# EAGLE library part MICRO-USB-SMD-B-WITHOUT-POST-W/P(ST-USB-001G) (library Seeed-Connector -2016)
320010000
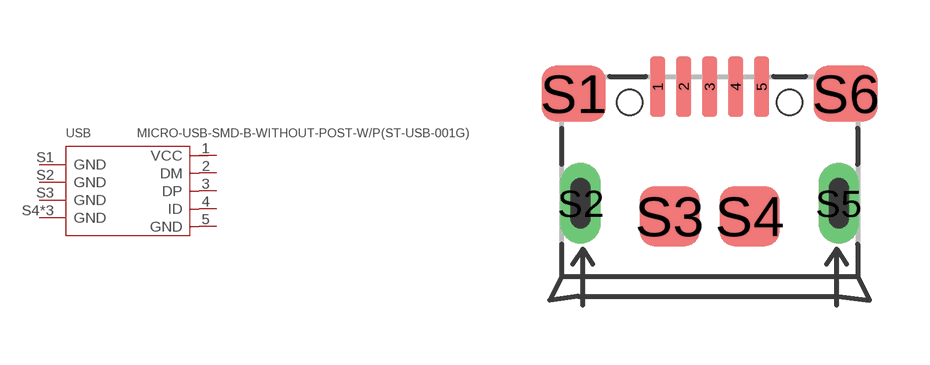
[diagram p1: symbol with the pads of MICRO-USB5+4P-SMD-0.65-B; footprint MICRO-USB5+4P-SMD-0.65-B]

Designator prefix USB

## MICRO-USB-SMD-B-WITHOUT-POST-W/P(ST-USB-001G) (MPN: ST-USB-001G; VALUE: ST-USB-001G)  [MICRO-USB5+4P-SMD-0.65-B]
1  VCC
2  DM
3  DP
4  ID
5  GND
S1  GND
S2  GND
S3  GND
S4  GND
S5  GND
S6  GND

## Footprint MICRO-USB5+4P-SMD-0.65-B (pad centres in mm)
smd 0.381 x 1.524: 1 -1.3,-0.25; 2 -0.65,-0.25; 3 0,-0.25; 4 0.65,-0.25; 5 1.3,-0.25
smd 1.6 x 1.397: S1 -3.4,-0.427; S6 3.4,-0.427
drill 0.508 pad 1.016 long: S2 -3.226,-3.175; S5 3.226,-3.175
smd 1.5 x 1.5: S3 -1,-3.5; S4 1,-3.5
hole 0.635 at -2,-0.65
hole 0.635 at 2,-0.65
